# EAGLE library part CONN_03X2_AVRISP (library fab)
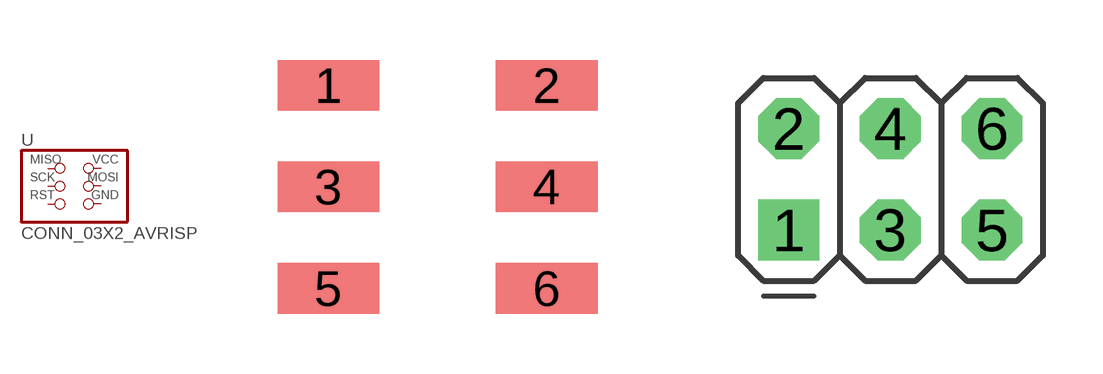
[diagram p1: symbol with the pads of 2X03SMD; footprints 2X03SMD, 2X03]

Designator prefix -

## CONN_03X2_AVRISPSMD  [2X03SMD]
1  MISO  pas
2  VCC  pas
3  SCK  pas
4  MOSI  pas
5  RST  pas
6  GND  pas

## CONN_03X2_AVRISP  [2X03]
Pads as for 2X03SMD

## Footprint 2X03SMD (pad centres in mm)
smd 2.54 x 1.27: 1 -2.54,2.54; 2 2.92,2.54; 3 -2.54,0; 4 2.92,0; 5 -2.54,-2.54; 6 2.92,-2.54

## Footprint 2X03 (pad centres in mm)
PIN HEADER
drill 1.016 square: 1 -2.54,-1.27
drill 1.016 octagon: 2 -2.54,1.27; 3 0,-1.27; 4 0,1.27; 5 2.54,-1.27; 6 2.54,1.27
